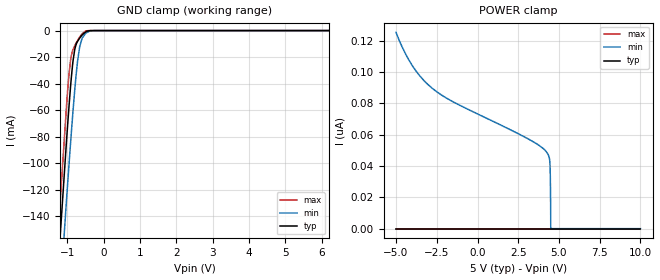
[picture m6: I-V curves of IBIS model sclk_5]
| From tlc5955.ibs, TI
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|   sclk_5 Model
[Model]   sclk_5
Model_type   Input
Vinl = 1.5
Vinh = 3.5
|   typ   min   max
|   (nom PVT)   (fast PVT)   (slow PVT)
C_comp   1.384e-12   1.346e-12   1.437e-12
[Model spec]
|subparameter
Vinl   1.5   1.35   1.65
Vinh   3.5   3.15   3.85
| Where nom  PVT is Nominal Process, 5V, 27C
|   Fast PVT is Strong Process,  5.5V, -40C
|   Slow PVT is Weak Process,   4.5V, 125C
[Voltage Range]   5   4.5   5.5
|Junction Temperature
[Temperature Range]   27   125   -40
[Power Clamp Reference]   5   4.5   5.5
[GND Clamp Reference]   0   0   0
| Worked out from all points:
|   GND clamp passes 1 mA (typ) near -0.50 V on its own axis
[GND Clamp]
|   Voltage   I(typ)   I(min)   I(max)
-5V       -1.942A    -1.924A    -1.966A
-1.252V   -177.3mA   -220mA     -152.4mA
-1.19V    -151mA     -194.4mA   -125.3mA
-1.026V   -83.69mA   -128.2mA   -57.38mA
-952mV    -55.48mA   -99.25mA   -31.75mA
-915mV    -42.66mA   -85.33mA   -22.69mA
-846.5mV  -23.01mA   -60.72mA   -14.36mA
-750mV    -9.746mA   -30.51mA   -8.867mA
-662mV    -5.628mA   -12.12mA   -4.842mA
-594.5mV  -3.34mA    -5.65mA    -2.395mA
-500mV    -1.061mA   -2.201mA   -419.1uA
10V       0A         0A         0A
[POWER Clamp]
|   Voltage   I(typ)   I(min)   I(max)
-5V       0A         125.2nA    0A
-3.992V   0A         103.8nA    0A
-2.785V   0A         89.59nA    0A
3.095V    0A         57.32nA    0A
4.212V    0A         49.21nA    0A
4.364V    0A         46.52nA    0A
4.441V    0A         42.18nA    0A
4.459V    0A         37.17nA    0A
4.473V    0A         29.29nA    0A
4.49V     0A         10.96nA    0A
4.495V    0A         0A         0A
10V       0A         0A         0A
